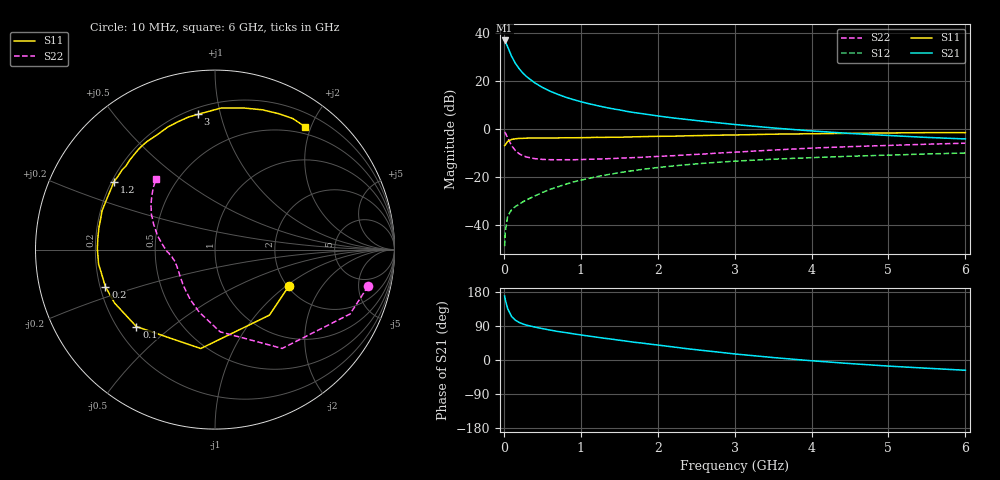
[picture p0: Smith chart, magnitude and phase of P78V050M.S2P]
! SIEMENS Small Signal Semiconductors
! BFP196
! Si NPN RF Bipolar Junction Transistor in SOT143
! VCE = 8 V  IC = 50 mA
! Common Emitter S-Parameters:  May  1996
# GHz  S  MA  R  50
!  f  S11  S21  S12  S22
! GHz  MAG  ANG  MAG  ANG  MAG  ANG  MAG  ANG
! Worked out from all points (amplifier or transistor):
!   36 points, 10 MHz to 6 GHz, reference 50 ohm
!   highest |S21| = 36.9 dB at 10 MHz (marker M1)
!   |S21| within 3 dB of that: start of sweep to 53.93 MHz
!   unconditionally stable (mu >= 1): 500.3 MHz to 4.574 GHz
!   at 250 MHz: K = 0.79, MSG = 26.7 dB, |S12| = -30.1 dB
!   at 1.4 GHz: K = 1.09, MAG = 11.8 dB, |S12| = -18.6 dB
!   at 6 GHz: K = 0.98, MSG = 2.9 dB, |S12| = -9.9 dB
!   S11 on the Smith chart (normalised r, x): 10 MHz: 2.03, -1.05; 100 MHz: 0.28, -0.38; 200 MHz: 0.22, -0.16; 1.2 GHz: 0.21, +0.29; 3 GHz: 0.24, +0.85; 6 GHz: 0.39, +1.91
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0.01  0.4589 -26.5  70.18 168.9  0.0037 78.5  0.8771 -13.4
0.02  0.4746 -50.3  65.67 158.0  0.0077 71.7  0.8337 -25.5
0.05  0.557 -98.2  51.43 135.2  0.0156 56.8  0.6657 -55.8
0.1  0.6129 -135.6  33.12 115.1  0.0212 47.1  0.459 -86.4
0.15  0.6336 -151.9  23.49 105.0  0.0247 47.3  0.3594 -104.2
0.2  0.6447 -161.4  18.11 99.0  0.0275 48.6  0.3094 -116.6
0.25  0.6467 -168.5  14.55 94.9  0.0311 50.4  0.2787 -126.2
0.3  0.6536 -172.9  12.24 91.7  0.0342 53.8  0.2637 -132.6
0.4  0.6555 179.6  9.272 87.0  0.0408 57.0  0.2446 -142.8
0.5  0.6558 174.5  7.425 82.9  0.0482 58.6  0.236 -149.5
0.6  0.6583 169.3  6.203 79.0  0.0562 60.1  0.2328 -154.0
0.7  0.66 164.7  5.328 75.3  0.0633 60.4  0.2317 -157.6
0.9  0.6647 157.1  4.151 69.2  0.0798 59.7  0.232 -162.9
1.1  0.6706 149.8  3.414 63.2  0.0947 58.6  0.2372 -166.5
1.2  0.6787 146.2  3.135 60.5  0.1025 57.6  0.2397 -168.1
1.7  0.6952 130.3  2.214 46.7  0.139 51.5  0.2571 -175.5
2.2  0.7159 116.8  1.718 34.5  0.1723 44.4  0.2814 177.9
3  0.7596 97.2  1.256 16.0  0.2169 32.9  0.3332 165.3
3.5  0.7896 87.5  1.064 6.5  0.2381 26.0  0.3691 157.7
4.5  0.8224 71.3  0.817 -9.4  0.2743 14.3  0.4347 145.1
5.5  0.8492 59.3  0.676 -21.7  0.3057 3.7  0.4879 134.8
6  0.8489 53.7  0.628 -27.1  0.3208 -1.8  0.5129 129.7
